|Texas Instruments Incorporated
|tmux5509,  2 data line 4:1 Mux
[IBIS Ver]   4.1
[File name]   tmux5509.ibs
[Date]   06/29/26
[File Rev]   1.0
[Source]
| Texas Instruments Incorporated.
| ASC-INT-MUX
| 12500 TI Blvd
| Dallas, TX - 75243
[Notes]   Revision History:
| Rev 1.0: 06/29/26
| - Initial version of the model
| - Model generated from simulations in SPECTRE
| - C_comp although listed in numerical order of value are
|   obtained from varying PVT conditions. For PVT conditions for
|   each specific value refer the buffer description under
|   respective [Model]. IBIS model user is responsible for using
|   appropriate C_comp to simulate for Signal Integrity.
[Disclaimer]
| This model is designed as an aid for customers of Texas Instruments.
| TI and its licensors and suppliers make no warranties, either expressed
| or implied, with respect to this  model, including the warranties of
| merchantability or fitness for a particular purpose. The model is
| provided solely on an "as is" basis. The entire risk as to its quality
| and performance is with the customer.
| This model is subject to change without notice. Texas Instruments
| Incorporated is not responsible for updating this model.
[Copyright]
(C) Copyright 2026 Texas Instruments Incorporated.All rights reserved.
|  Component TMUX5509D 16-pin - D package
|  Part # TMUX5509D
[Component]   TMUX5509D
[Manufacturer]  TI
[Package]
|   typ   min   max
R_pkg   0.075   NA   NA
L_pkg   1nH   NA   NA
C_pkg   0.25pF   NA   NA
[Pin]   signal_name   model_name
   1   A0   inbuf
   2   EN   inbuf
   3   VSS   power
   4   S1A   sterm
   5   S2A   sterm
   6   S3A   sterm
   7   S4A   sterm
   8   DA   dterm
   9   DB   dterm
   10   S4B   sterm
   11   S3B   sterm
   12   S2B   sterm
   13   S1B   sterm
   14   VDD   power
   15   GND   gnd
   16   A1   inbuf
[Series Switch Groups]
On 1 /
On 2 /
On 3 /
On 4 /
Off 1 /
[Series Pin Mapping]  pin_2 model_name function_table_group
   4   8   switch_dual_20   1
   5   8   switch_dual_20   1
   6   8   switch_dual_20   1
   7   8   switch_dual_20   1
  13   9   switch_dual_20   1
  12   9   switch_dual_20   1
  11   9   switch_dual_20   1
  10   9   switch_dual_20   1
|   4   8   switch_dual_15   1
|   5   8   switch_dual_15   1
|   6   8   switch_dual_15   1
|   7   8   switch_dual_15   1
|  13   9   switch_dual_15   1
|  12   9   switch_dual_15   1
|  11   9   switch_dual_15   1
|  10   9   switch_dual_15   1
|   4   8   switch_40   1
|   5   8   switch_40   1
|   6   8   switch_40   1
|   7   8   switch_40   1
|  13   9   switch_40   1
|  12   9   switch_40   1
|  11   9   switch_40   1
|  10   9   switch_40   1
|   4   8   switch_12   1
|   5   8   switch_12   1
|   6   8   switch_12   1
|   7   8   switch_12   1
|  13   9   switch_12   1
|  12   9   switch_12   1
|  11   9   switch_12   1
|  10   9   switch_12   1
|   4   8   switch_5   1
|   5   8   switch_5   1
|   6   8   switch_5   1
|   7   8   switch_5   1
|  13   9   switch_5   1
|  12   9   switch_5   1
|  11   9   switch_5   1
|  10   9   switch_5   1
|  Component TMUX5509PW 16-pin - PW package
|  Part # TMUX5509PW
[Component]   TMUX5509PW
[Manufacturer]  TI
[Package]
|   typ   min   max
R_pkg   0.075   NA   NA
L_pkg   1nH   NA   NA
C_pkg   0.25pF   NA   NA
[Pin]   signal_name   model_name
   1   A0   inbuf
   2   EN   inbuf
   3   VSS   power
   4   S1A   sterm
   5   S2A   sterm
   6   S3A   sterm
   7   S4A   sterm
   8   DA   dterm
   9   DB   dterm
   10   S4B   sterm
   11   S3B   sterm
   12   S2B   sterm
   13   S1B   sterm
   14   VDD   power
   15   GND   gnd
   16   A1   inbuf
[Series Switch Groups]
On 1 /
On 2 /
On 3 /
On 4 /
Off 1 /
[Series Pin Mapping]  pin_2 model_name function_table_group
   4   8   switch_dual_20   1
   5   8   switch_dual_20   1
   6   8   switch_dual_20   1
   7   8   switch_dual_20   1
  13   9   switch_dual_20   1
  12   9   switch_dual_20   1
  11   9   switch_dual_20   1
  10   9   switch_dual_20   1
|   4   8   switch_dual_15   1
|   5   8   switch_dual_15   1
|   6   8   switch_dual_15   1
|   7   8   switch_dual_15   1
|  13   9   switch_dual_15   1
|  12   9   switch_dual_15   1
|  11   9   switch_dual_15   1
|  10   9   switch_dual_15   1
|   4   8   switch_40   1
|   5   8   switch_40   1
|   6   8   switch_40   1
|   7   8   switch_40   1
|  13   9   switch_40   1
|  12   9   switch_40   1
|  11   9   switch_40   1
|  10   9   switch_40   1
|   4   8   switch_12   1
|   5   8   switch_12   1
|   6   8   switch_12   1
|   7   8   switch_12   1
|  13   9   switch_12   1
|  12   9   switch_12   1
|  11   9   switch_12   1
|  10   9   switch_12   1
|   4   8   switch_5   1
|   5   8   switch_5   1
|   6   8   switch_5   1
|   7   8   switch_5   1
|  13   9   switch_5   1
|  12   9   switch_5   1
|  11   9   switch_5   1
|  10   9   switch_5   1
|  Component TMUX5509RSV 16-pin - RSV package
|  Part # TMUX5509RSV
[Component]   TMUX5509RSV
[Manufacturer]  TI
[Package]
|   typ   min   max
R_pkg   0.075   NA   NA
L_pkg   1nH   NA   NA
C_pkg   0.25pF   NA   NA
[Pin]   signal_name   model_name
   1   A0   inbuf
   2   EN   inbuf
   3   VSS   power
   4   S1A   sterm
   5   S2A   sterm
   6   S3A   sterm
   7   S4A   sterm
   8   DA   dterm
   9   DB   dterm
   10   S4B   sterm
   11   S3B   sterm
   12   S2B   sterm
   13   S1B   sterm
   14   VDD   power
   15   GND   gnd
   16   A1   inbuf
[Series Switch Groups]
On 1 /
On 2 /
On 3 /
On 4 /
Off 1 /
[Series Pin Mapping]  pin_2 model_name function_table_group
   4   8   switch_dual_20   1
   5   8   switch_dual_20   1
   6   8   switch_dual_20   1
   7   8   switch_dual_20   1
  13   9   switch_dual_20   1
  12   9   switch_dual_20   1
  11   9   switch_dual_20   1
  10   9   switch_dual_20   1
|   4   8   switch_dual_15   1
|   5   8   switch_dual_15   1
|   6   8   switch_dual_15   1
|   7   8   switch_dual_15   1
|  13   9   switch_dual_15   1
|  12   9   switch_dual_15   1
|  11   9   switch_dual_15   1
|  10   9   switch_dual_15   1
|   4   8   switch_40   1
|   5   8   switch_40   1
|   6   8   switch_40   1
|   7   8   switch_40   1
|  13   9   switch_40   1
|  12   9   switch_40   1
|  11   9   switch_40   1
|  10   9   switch_40   1
|   4   8   switch_12   1
|   5   8   switch_12   1
|   6   8   switch_12   1
|   7   8   switch_12   1
|  13   9   switch_12   1
|  12   9   switch_12   1
|  11   9   switch_12   1
|  10   9   switch_12   1
|   4   8   switch_5   1
|   5   8   switch_5   1
|   6   8   switch_5   1
|   7   8   switch_5   1
|  13   9   switch_5   1
|  12   9   switch_5   1
|  11   9   switch_5   1
|  10   9   switch_5   1
[Model Selector] dterm
dterm_dual_20 Use for operation at +/-20V
dterm_dual_15 Use for operation at +/-15V
dterm_40 Use for operation at 40V
dterm_12 Use for operation at 12V
dterm_5 Use for operation at 5V
[Model Selector] sterm
sterm_dual_20 Use for operation at +/-20V
sterm_dual_15 Use for operation at +/-15V
sterm_40 Use for operation at 40V
sterm_12 Use for operation at 12V
sterm_5 Use for operation at 5V
[Model Selector] inbuf
inbuf_dual_20 Use for operation at +/-20V
inbuf_dual_15 Use for operation at +/-15V
inbuf_40 Use for operation at 40V
inbuf_12 Use for operation at 12V
inbuf_5 Use for operation at 5V
| switch_dual_20
[Model]   switch_dual_20
Model_type   Series_switch
|   typ   min   max
C_comp   2.533030e-12   NA   NA
[Voltage Range]   20   NA   NA
[Power Clamp Reference]   20   NA   NA
[Temperature Range]   27   NA   NA
[On]
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[Off]
|   typ   min   max
[R Series]   10G   NA   NA
| switch_dual_15
[Model]   switch_dual_15
Model_type   Series_switch
|   typ   min   max
C_comp   2.533030e-12   NA   NA
[Voltage Range]   15   NA   NA
[Power Clamp Reference]   15   NA   NA
[Temperature Range]   27   NA   NA
[On]
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[Off]
|   typ   min   max
[R Series]   10G   NA   NA
| switch_40
[Model]   switch_40
Model_type   Series_switch
|   typ   min   max
C_comp   2.533030e-12   NA   NA
[Voltage Range]   40   NA   NA
[Power Clamp Reference]   40   NA   NA
[Temperature Range]   27   NA   NA
[On]
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[Off]
|   typ   min   max
[R Series]   10G   NA   NA
| switch_12
[Model]   switch_12
Model_type   Series_switch
|   typ   min   max
C_comp   2.533030e-12   NA   NA
[Voltage Range]   12   NA   NA
[Power Clamp Reference]   12   NA   NA
[Temperature Range]   27   NA   NA
[On]
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[Off]
|   typ   min   max
[R Series]   10G   NA   NA
| switch_5
[Model]   switch_5
Model_type   Series_switch
|   typ   min   max
C_comp   2.533030e-12   NA   NA
[Voltage Range]   5   NA   NA
[Power Clamp Reference]   5   NA   NA
[Temperature Range]   27   NA   NA
[On]
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[Off]
|   typ   min   max
[R Series]   10G   NA   NA
| Models and submodels in the file (20): dterm_dual_20 (Terminator), dterm_dual_15 (Terminator), dterm_40 (Terminator), dterm_12 (Terminator), dterm_5 (Terminator), switch_dual_20 (Series_switch), switch_dual_15 (Series_switch), switch_40 (Series_switch), switch_12 (Series_switch), switch_5 (Series_switch), sterm_dual_20 (Terminator), sterm_dual_15 (Terminator), sterm_40 (Terminator), sterm_12 (Terminator), sterm_5 (Terminator), inbuf_dual_20 (Input), inbuf_dual_15 (Input), inbuf_40 (Input), inbuf_12 (Input), inbuf_5 (Input)
